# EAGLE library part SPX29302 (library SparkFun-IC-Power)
3A LDO regulator
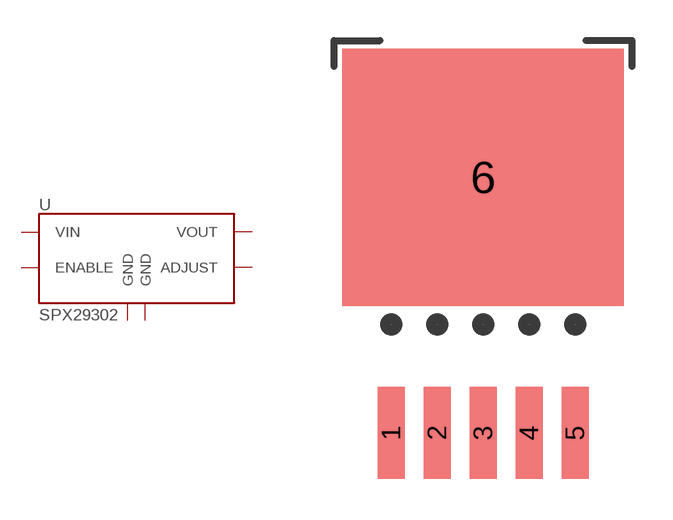
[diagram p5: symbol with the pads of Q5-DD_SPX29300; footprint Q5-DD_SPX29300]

Designator prefix U

## SPX29302 (PROD_ID: VREG-08337)  [Q5-DD_SPX29300]
1  ENABLE
2  VIN
3  GND
4  VOUT
5  ADJUST
6  GND

## Footprint Q5-DD_SPX29300 (pad centres in mm)
smd 1 x 3.4: 1 -3.4,-7.875; 2 -1.7,-7.875; 3 0,-7.875; 4 1.7,-7.875; 5 3.4,-7.875
smd 10.414 x 9.525: 6 0,1.595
